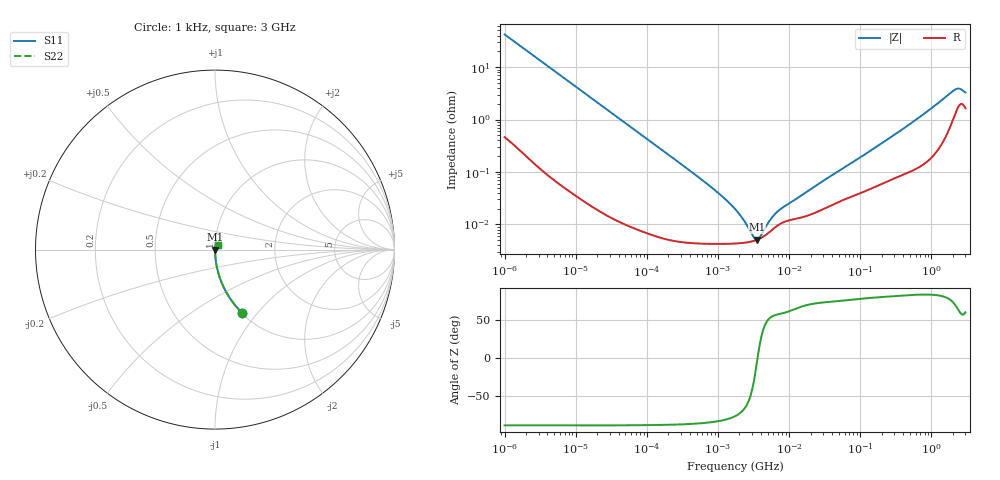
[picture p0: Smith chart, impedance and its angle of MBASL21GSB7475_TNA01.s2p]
! MBASL21GSB7475_TNA01  S-PARAMETER MODEL  ( Standard Model )
! Model Generated by TAIYO YUDEN Corporation (http://www.ty-top.com)
! Version 1.0
! TAIYO YUDEN Control No. 220601
! Copyright(c) 2013 TAIYO YUDEN CO.,LTD. All Rights Reserved.
! Product Description (link to TY-COMPAS)
! https://ds.yuden.co.jp/TYCOMPAS/or/detail?pn=MBASL21GSB7475KTNA01&u=M
! Products Name : Multilayer Ceramic Capacitors
! Characteristics :
!  Capacitance : 4.7 [uF] , Rated Voltage : 10 [V] , TCC : X7R
!  Case Size : 2.0 x 1.25 / 0.079 x 0.049 [mm/inch] , Thickness : 1.25 / 0.049 [mm/inch]
!  (Conditions: Temperature = 25 [degC] , DC Bias Voltage = 0 [V])
! External Node Assignments :
!  1  o---| |---o  2
! GND o---------o GND
! Frequency Range : 1kHz  -  3GHz  [ 401 STEP ]
# MHZ S RI R 50
! Freq[MHz].  S11 Real  S11 Imag  S21 Real  S21 Imag  S12 Real  S12 Imag  S22 Real  S22 Imag
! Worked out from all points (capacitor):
!   401 points, 1 kHz to 3 GHz, reference 50 ohm
!   read as one part in series: C = 3.78 uF near 1.077 kHz
!   lowest |Z| = 5.12 mohm at 3.517 MHz (marker M1)
!   series resonance near 3.598 MHz, so ESL is about 520 pH
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0.001  0.1526 -0.3542  0.8474 0.3542  0.8474 0.3542  0.1526 -0.3542
0.001685  0.061 -0.2344  0.939 0.2344  0.939 0.2344  0.061 -0.2344
0.003177  0.0185 -0.1306  0.9815 0.1306  0.9815 0.1306  0.0185 -0.1306
0.005768  0.00597 -0.0731  0.994 0.0731  0.994 0.0731  0.00597 -0.0731
0.01216  0.00152 -0.0349  0.9985 0.0349  0.9985 0.0349  0.00152 -0.0349
0.147855  6.52e-05 -0.00291  0.9999 0.00291  0.9999 0.00291  6.52e-05 -0.00291
0.791611  4.29e-05 -0.00052  1 0.00052  1 0.00052  4.29e-05 -0.00052
1.238299  4.27e-05 -0.000309  1 0.000309  1 0.000309  4.27e-05 -0.000309
1.732051  4.32e-05 -0.000193  1 0.000193  1 0.000193  4.32e-05 -0.000193
2.514714  4.53e-05 -8.89e-05  1 8.89e-05  1 8.89e-05  4.53e-05 -8.89e-05
2.709407  4.61e-05 -6.99e-05  1 6.99e-05  1 6.99e-05  4.61e-05 -6.99e-05
3.517417  5.09e-05 -5.48e-06  0.9999 5.48e-06  0.9999 5.48e-06  5.09e-05 -5.48e-06
4.566395  6.15e-05 5.78e-05  0.9999 -5.78e-05  0.9999 -5.78e-05  6.15e-05 5.78e-05
4.919932  6.63e-05 7.56e-05  0.9999 -7.56e-05  0.9999 -7.56e-05  6.63e-05 7.56e-05
6.153411  8.49e-05 0.000126  0.9999 -0.000126  0.9999 -0.000126  8.49e-05 0.000126
7.414467  0.000102 0.000163  0.9999 -0.000163  0.9999 -0.000163  0.000102 0.000163
21.06097  0.000159 0.000466  0.9998 -0.000466  0.9998 -0.000466  0.000159 0.000466
256.0921  0.000706 0.00437  0.9993 -0.00437  0.9993 -0.00437  0.000706 0.00437
727.4359  0.00146 0.0118  0.9985 -0.0118  0.9985 -0.0118  0.00146 0.0118
2066.299  0.0121 0.0335  0.9879 -0.0335  0.9879 -0.0335  0.0121 0.0335
2398.636  0.0186 0.0336  0.9814 -0.0336  0.9814 -0.0336  0.0186 0.0336
3000  0.0169 0.0276  0.9831 -0.0276  0.9831 -0.0276  0.0169 0.0276
